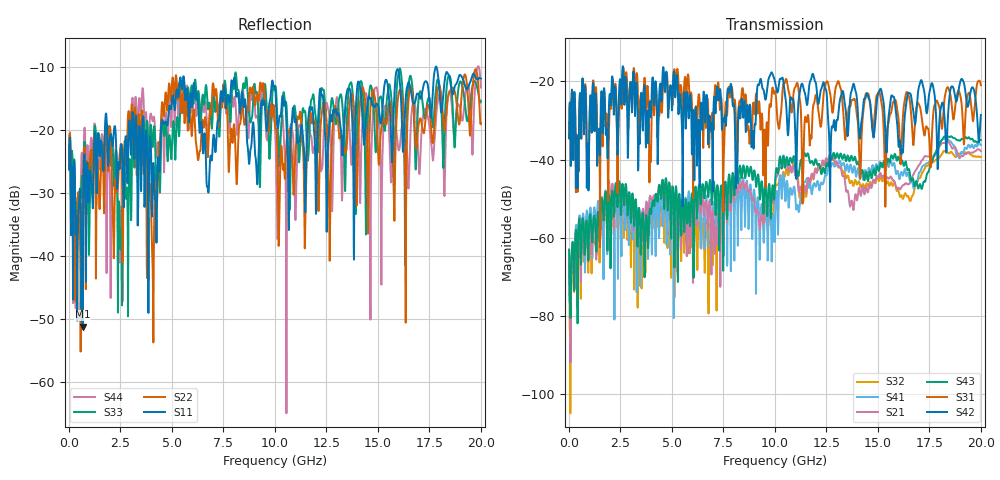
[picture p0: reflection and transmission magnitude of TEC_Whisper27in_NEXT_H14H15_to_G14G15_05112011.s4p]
! Tyco Electronics
! H14F15-H14G15_NEXT
!! PART DESCRIPTION: Whisper 27in Megtron 6 VLP-HVLP-VLP Channel Model, bulkhead 2.4mm test pts
!! MODEL DESCRIPTION: System 4-port S-parameter
!! MODEL STATUS: Measured
!! MODEL GEOMETRY: Channel Model
!! MODEL FREQUENCY RANGE: DC to 20.000 GHz in 10.000 MHz frequency steps
!! MODEL EDGE RATE LIMITATION: 25.00 ps (Using conservative 0.5/Fmax rule of thumb)
!! TIME-DOMAIN TRANSFORM CAUTIONS:
!! 1.) Do not simulate transient edge rates faster than the number listed above.  Edge rates faster than this number
!!  contain significant spectral content at frequencies above the model's highest frequency.
!! 2.) Even when simulating edge rates that are slower than the number listed above, be aware that the best time
!!  resolution possible with a direct iFFT is (1 / 2Fmax).  As a result, time resolution is typically not adequate
!!  for most time-domain simulations unless tricks such as windowing are used to minimize leakage and aliasing.
!! 3.) Because the model has a uniform frequency step, a direct iFFT will result in an impulse that that has a time
!!  length given by either (1 / Fstep) or (1 / 2Fstep), depending on the transform being used.  Care has been taken
!!  in selecting the frequency step to ensure a settled impulse response for the model.  Therefore, convolution with
!!  the model's impulse response should present no issues.  However, if directly concatenating s-parameter models
!!  in the frequency domain a user must either interpolate necessary interim frequencies or complete impulse response
!!  zero-padding.  Impulse response zero-padding is more difficult, but more accurate.
!! PORT DEFINITIONS:
!! Port  1  ----->  Side A  H14  G14  Side A  <-----  Port  2
!! Port  3  ----->  Side A  H15  G15  Side A  <-----  Port  4
! Point-to-Point link (differential)  !
! Connectors:  !
!  1: STRADA Whisper  !
! Materials:  !
!  Backplane: Megtron-6 HVLP  !
!  Daughtercard: Megtron-6 VLP  !
! Stack-up:  !
!  Backplane: 20 layers, 200mil thick  !
!  Daughtercard: 14 layers, 110mil thick  !
! Trace Length:  !
!  Backplane: 17in  !
!  Daightercards: 5in  !
! Trace Width:  !
!  Backplane: 8-13-8 mils  !
!  Daughtercards: 6-9-6 mils  !
! Geometry:  !
!  Backplane: Stripline  !
!  Daughtercards: Stripline  !
! Freq. Range: 0 GHz - 20 GHz  !
! Note1: non-mixed-mode s-parameters  !
! Note2: channel includes 2.4mm test points  !
! Created Wed May 11 15:03:07 2011
! 4 Port Network Data from SP1.SP block
! freq  magS11  angS11  magS12  angS12  magS13  angS13  magS14  angS14
!  magS21  angS21  magS22  angS22  magS23  angS23  magS24  angS24
!  magS31  angS31  magS32  angS32  magS33  angS33  magS34  angS34
!  magS41  angS41  magS42  angS42  magS43  angS43  magS44  angS44
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# hz S ma R 50
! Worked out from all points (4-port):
!   2000 points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, 10 MHz to 20 GHz, reference 50 ohm
!   strongest paths, dB at 10 MHz, 5.01 GHz, 10.01 GHz, 15.01 GHz, 20 GHz:
!     S42: -34.5, -27.3, -20.2, -23.2, -28.6
!     S31: -34.6, -25.5, -22.5, -23.0, -21.0
!     S43: -63.1, -47.9, -45.9, -42.2, -35.0
!     S21: -62.9, -47.0, -46.3, -44.7, -37.8
!     S41: -66.9, -49.0, -54.8, -42.5, -36.2
!     S32: -66.8, -51.8, -47.5, -44.9, -39.3
!   lowest |S11| = -51.2 dB at 660 MHz (marker M1), VSWR 1.01, Z = 50.1 - j0.261 ohm
!   |S11| at or under -10 dB: start of sweep to 17.81 GHz; 17.84 GHz to end of sweep
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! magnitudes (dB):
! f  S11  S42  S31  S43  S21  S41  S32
! 10 MHz  -26.2  -34.5  -34.6  -63.1  -62.9  -66.9  -66.8
! 660 MHz  -51.2  -19.2  -19.4  -55.2  -55.0  -55.0  -58.6
! 2.53 GHz  -22.6  -24.3  -23.2  -53.9  -51.8  -56.5  -56.9
! 2.98 GHz  -21.0  -20.4  -20.3  -52.2  -52.5  -51.2  -55.1
! 4.07 GHz  -27.3  -19.0  -22.7  -50.6  -50.1  -53.2  -54.0
! 5.12 GHz  -16.6  -18.7  -16.9  -67.5  -57.4  -55.2  -75.3
! 20 GHz  -11.9  -28.6  -21.0  -35.0  -37.8  -36.2  -39.3
